FUNCTION_BLOCK FB 15
TITLE =
VERSION : 0.1


VAR_INPUT
  T1_2 : BOOL ;
  T2_3 : BOOL  := TRUE;
  T3_4 : BOOL  := TRUE;
  T4_5 : BOOL  := TRUE;
  T5_6 : BOOL  := TRUE;
  T6_7 : BOOL  := TRUE;
  T7_8 : BOOL  := TRUE;
  T8_9 : BOOL  := TRUE;
  T9_10 : BOOL  := TRUE;
  T10_1 : BOOL  := TRUE;
  RESET : BOOL ;
END_VAR
VAR_OUTPUT
  SR : INT ;
END_VAR
VAR
  SRO_1 : BOOL  := TRUE;
  SRO_2 : BOOL ;
  SRO_3 : BOOL ;
  SRO_4 : BOOL ;
  SRO_5 : BOOL ;
  SRO_6 : BOOL ;
  SRO_7 : BOOL ;
  SRO_8 : BOOL ;
  SRO_9 : BOOL ;
  SRO_10 : BOOL ;
END_VAR
BEGIN
NETWORK
TITLE =



      U(    ;
      U(    ;
      O     #RESET;
      O     ;
      U     #SRO_10;
      U     #T10_1;
      )     ;
      S     #SRO_1;
      U     #SRO_2;
      R     #SRO_1;
      U     #SRO_1;
      )     ;
      SPBNB _001;
      L     1;
      T     #SR;
_001: NOP   0;
NETWORK
TITLE =

      U(    ;
      U     #SRO_1;
      U     #T1_2;
      S     #SRO_2;
      U(    ;
      O     #SRO_3;
      O     #RESET;
      )     ;
      R     #SRO_2;
      U     #SRO_2;
      )     ;
      SPBNB _002;
      L     2;
      T     #SR;
_002: NOP   0;
NETWORK
TITLE =

      U(    ;
      U     #SRO_2;
      U     #T2_3;
      S     #SRO_3;
      U(    ;
      O     #SRO_4;
      O     #RESET;
      )     ;
      R     #SRO_3;
      U     #SRO_3;
      )     ;
      SPBNB _003;
      L     3;
      T     #SR;
_003: NOP   0;
NETWORK
TITLE =

      U(    ;
      U     #SRO_3;
      U     #T3_4;
      S     #SRO_4;
      U(    ;
      O     #SRO_5;
      O     #RESET;
      )     ;
      R     #SRO_4;
      U     #SRO_4;
      )     ;
      SPBNB _004;
      L     4;
      T     #SR;
_004: NOP   0;
NETWORK
TITLE =

      U(    ;
      U     #SRO_4;
      U     #T4_5;
      S     #SRO_5;
      U(    ;
      O     #SRO_6;
      O     #RESET;
      )     ;
      R     #SRO_5;
      U     #SRO_5;
      )     ;
      SPBNB _005;
      L     5;
      T     #SR;
_005: NOP   0;
NETWORK
TITLE =

      U(    ;
      U     #SRO_5;
      U     #T5_6;
      S     #SRO_6;
      U(    ;
      O     #SRO_7;
      O     #RESET;
      )     ;
      R     #SRO_6;
      U     #SRO_6;
      )     ;
      SPBNB _006;
      L     6;
      T     #SR;
_006: NOP   0;
NETWORK
TITLE =

      U(    ;
      U     #SRO_6;
      U     #T6_7;
      S     #SRO_7;
      U(    ;
      O     #SRO_8;
      O     #RESET;
      )     ;
      R     #SRO_7;
      U     #SRO_7;
      )     ;
      SPBNB _007;
      L     7;
      T     #SR;
_007: NOP   0;
NETWORK
TITLE =

      U(    ;
      U     #SRO_7;
      U     #T7_8;
      S     #SRO_8;
      U(    ;
      O     #SRO_9;
      O     #RESET;
      )     ;
      R     #SRO_8;
      U     #SRO_8;
      )     ;
      SPBNB _008;
      L     8;
      T     #SR;
_008: NOP   0;
NETWORK
TITLE =

      U(    ;
      U     #SRO_8;
      U     #T8_9;
      S     #SRO_9;
      U(    ;
      O     #SRO_10;
      O     #RESET;
      )     ;
      R     #SRO_9;
      U     #SRO_9;
      )     ;
      SPBNB _009;
      L     9;
      T     #SR;
_009: NOP   0;
NETWORK
TITLE =

      U(    ;
      U     #SRO_9;
      U     #T9_10;
      S     #SRO_10;
      U(    ;
      O     #SRO_1;
      O     #RESET;
      )     ;
      R     #SRO_10;
      U     #SRO_10;
      )     ;
      SPBNB _00a;
      L     10;
      T     #SR;
_00a: NOP   0;
END_FUNCTION_BLOCK

FUNCTION FC 16 : VOID
TITLE =
VERSION : 0.1


VAR_INPUT
  SR : INT ;
  Zeit : TIMER ;
  Zeitw : S5TIME ;
  RESET : BOOL ;
END_VAR
VAR_OUTPUT
  _1Y1 : BOOL ;
  _2Y1 : BOOL ;
  _3Y1 : BOOL ;
  Y1 : BOOL ;
END_VAR
BEGIN
NETWORK
TITLE =
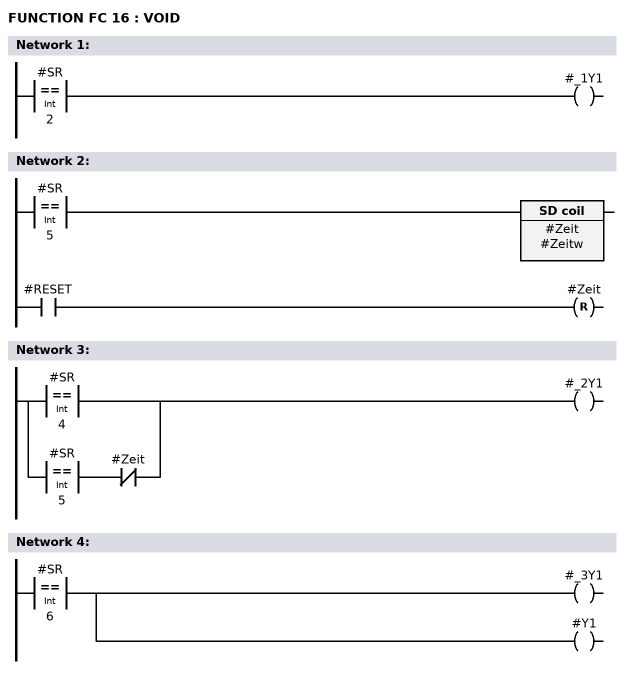
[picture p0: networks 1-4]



      L     #SR;
      L     2;
      ==I   ;
      =     #_1Y1;
NETWORK
TITLE =

      U(    ;
      L     #SR;
      L     5;
      ==I   ;
      )     ;
      L     #Zeitw;
      SE    #Zeit;
      U     #RESET;
      R     #Zeit;
      NOP   0;
      NOP   0;
      NOP   0;
NETWORK
TITLE =

      O(    ;
      L     #SR;
      L     4;
      ==I   ;
      )     ;
      O     ;
      U(    ;
      L     #SR;
      L     5;
      ==I   ;
      )     ;
      UN    #Zeit;
      =     #_2Y1;
NETWORK
TITLE =

      L     #SR;
      L     6;
      ==I   ;
      =     #_3Y1;
      =     #Y1;
END_FUNCTION

ORGANIZATION_BLOCK OB 1
TITLE = "Main Program Sweep (Cycle)"
VERSION : 0.1


VAR_TEMP
  OB1_EV_CLASS : BYTE ;	//Bits 0-3 = 1 (Coming event), Bits 4-7 = 1 (Event class 1)
  OB1_SCAN_1 : BYTE ;	//1 (Cold restart scan 1 of OB 1), 3 (Scan 2-n of OB 1)
  OB1_PRIORITY : BYTE ;	//Priority of OB Execution
  OB1_OB_NUMBR : BYTE ;	//1 (Organization block 1, OB1)
  OB1_RESERVED_1 : BYTE ;	//Reserved for system
  OB1_RESERVED_2 : BYTE ;	//Reserved for system
  OB1_PREV_CYCLE : INT ;	//Cycle time of previous OB1 scan (milliseconds)
  OB1_MIN_CYCLE : INT ;	//Minimum cycle time of OB1 (milliseconds)
  OB1_MAX_CYCLE : INT ;	//Maximum cycle time of OB1 (milliseconds)
  OB1_DATE_TIME : DATE_AND_TIME ;	//Date and time OB1 started
  Schritt : INT ;
END_VAR
BEGIN
NETWORK
TITLE =
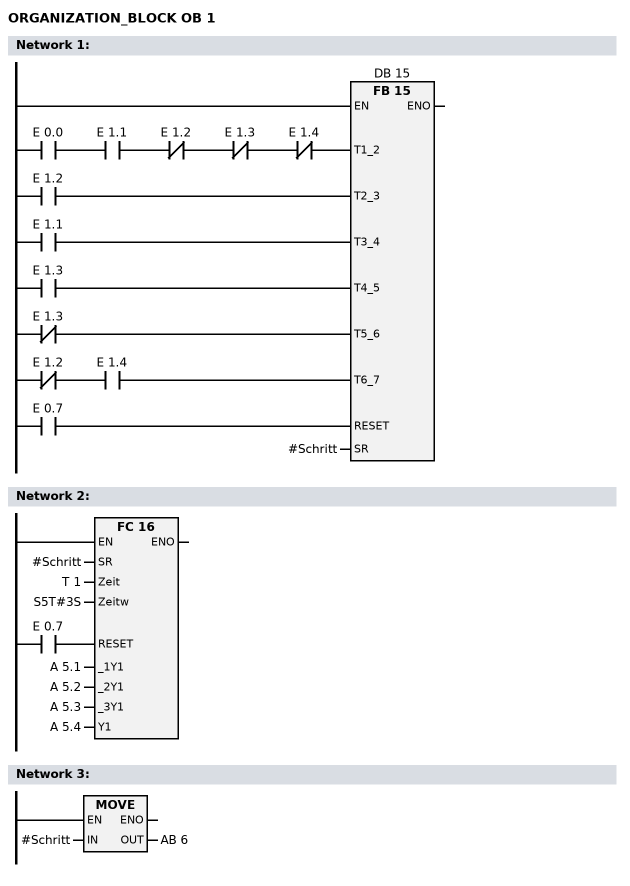
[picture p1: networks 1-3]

      U     E      0.0;
      U     E      1.1;
      UN    E      1.2;
      UN    E      1.3;
      UN    E      1.4;
      =     L     22.0;
      BLD   103;
      U     E      1.2;
      =     L     22.1;
      BLD   103;
      U     E      1.1;
      =     L     22.2;
      BLD   103;
      U     E      1.3;
      =     L     22.3;
      BLD   103;
      UN    E      1.3;
      =     L     22.4;
      BLD   103;
      UN    E      1.2;
      U     E      1.4;
      =     L     22.5;
      BLD   103;
      U     E      0.7;
      =     L     23.2;
      BLD   103;
      CALL FB    15 , DB    15 (
           T1_2                     := L     22.0,
           T2_3                     := L     22.1,
           T3_4                     := L     22.2,
           T4_5                     := L     22.3,
           T5_6                     := L     22.4,
           T6_7                     := L     22.5,
           RESET                    := L     23.2,
           SR                       := #Schritt);
      NOP   0;
NETWORK
TITLE =

      U     E      0.7;
      =     L     22.0;
      BLD   103;
      CALL FC    16 (
           SR                       := #Schritt,
           Zeit                     := T      1,
           Zeitw                    := S5T#3S,
           RESET                    := L     22.0,
           _1Y1                     := A      5.1,
           _2Y1                     := A      5.2,
           _3Y1                     := A      5.3,
           Y1                       := A      5.4);
      NOP   0;
NETWORK
TITLE =

      L     #Schritt;
      T     AB     6;
      NOP   0;
END_ORGANIZATION_BLOCK

